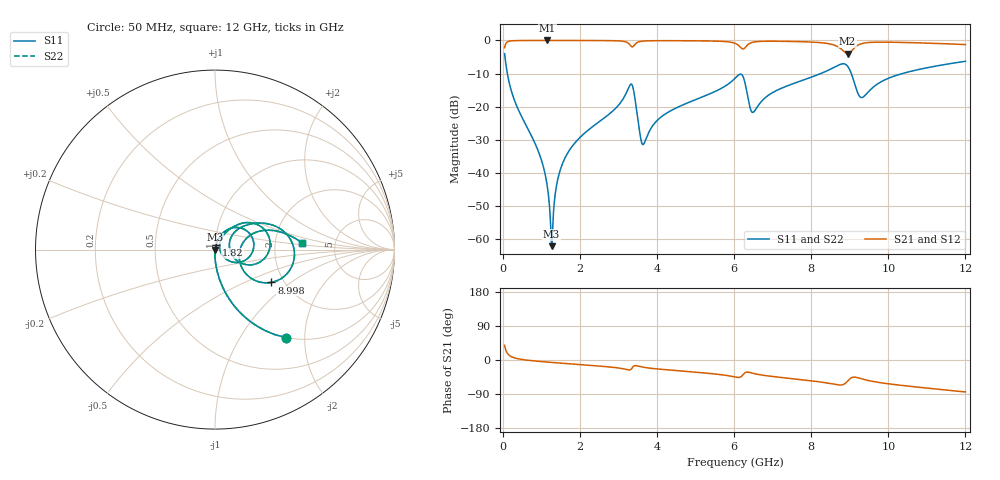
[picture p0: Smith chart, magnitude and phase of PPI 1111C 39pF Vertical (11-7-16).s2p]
# GHz S MA R 50
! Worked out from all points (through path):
!   1601 points, 50 MHz to 12 GHz, reference 50 ohm
!   highest |S21| = -0.01 dB at 1.155 GHz (marker M1); lowest = -4.0 dB at 8.945 GHz (marker M2)
!   group delay of S21, straight-line fit = 19.3 ps
!   lowest |S11| = -62.2 dB at 1.267 GHz (marker M3), VSWR 1.00, Z = 50.1 - j0.0248 ohm
!   |S11| at or under -10 dB: 120.9 MHz to 8.25 GHz (8.129 GHz wide, 194 % of centre); 9.041 GHz to 10.37 GHz (1.325 GHz wide, 13.7 % of centre)
!   |S22| runs from -62.2 to -4.0 dB; largest |S21 - S12| = 0
!   S11 on the Smith chart (normalised r, x): 50 MHz: 0.99, -1.62; 1.82 GHz: 1.01, +0.05; 8.998 GHz: 1.72, -0.73; 12 GHz: 2.84, +0.29
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0.05  0.6301 -51.2  0.7763 38.8  0.7763 38.8  0.6301 -51.2
0.2367188  0.1637 -81.6  0.9861 8.2  0.9861 8.2  0.1637 -81.6
0.9387813  0.02011 -91.7  0.9991 -3.6  0.9991 -3.6  0.02011 -91.7
1.155375  0.006347 -88.9  0.9992 -5.5  0.9992 -5.5  0.006347 -88.9
1.267406  0.0007793 -18.6  0.9992 -6.4  0.9992 -6.4  0.0007793 -18.6
1.469062  0.009927 77.2  0.999 -8.0  0.999 -8.0  0.009927 77.2
1.820094  0.02592 77.2  0.9986 -10.7  0.9986 -10.7  0.02592 77.2
2.044156  0.036 75.8  0.9981 -12.4  0.9981 -12.4  0.036 75.8
3.313844  0.2164 20.5  0.8374 -25.6  0.8374 -25.6  0.2164 20.5
3.396  0.1749 -20.5  0.8253 -16.3  0.8253 -16.3  0.1749 -20.5
3.627531  0.02683 5.1  0.9752 -18.8  0.9752 -18.8  0.02683 5.1
4.038312  0.06435 60.0  0.9908 -23.8  0.9908 -23.8  0.06435 60.0
6.025  0.2677 32.4  0.9055 -44.8  0.9055 -44.8  0.2677 32.4
6.219188  0.2947 -4.6  0.7459 -40.5  0.7459 -40.5  0.2947 -4.6
6.495531  0.08193 11.2  0.9414 -35.2  0.9414 -35.2  0.08193 11.2
8.019156  0.2806 31.8  0.9438 -55.0  0.9438 -55.0  0.2806 31.8
8.609188  0.3963 14.8  0.8457 -64.3  0.8457 -64.3  0.3963 14.8
8.945281  0.4083 -22.4  0.6331 -55.8  0.6331 -55.8  0.4083 -22.4
8.997563  0.3633 -30.2  0.6503 -50.2  0.6503 -50.2  0.3633 -30.2
9.303781  0.1371 -8.4  0.8921 -49.5  0.8921 -49.5  0.1371 -8.4
10.01331  0.2695 22.5  0.9412 -62.9  0.9412 -62.9  0.2695 22.5
12  0.4841 4.6  0.8658 -84.4  0.8658 -84.4  0.4841 4.6
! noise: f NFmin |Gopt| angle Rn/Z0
0.05  0.0003308  0.8511  0.8612  0.0004735
1.372  0.003262  0.634  6.902  0.001671
2.701  0.008566  0.7145  13.35  0.005846
4.031  0.01618  0.7704  20  0.01393
5.36  0.01777  0.7331  26.08  0.01262
6.682  0.03951  0.8444  32.6  0.04969
8.012  0.03356  0.7925  38.25  0.02984
9.341  0.0873  0.9041  44.47  0.171
10.67  0.03431  0.7525  49.19  0.02322
12  0.03072  0.7094  53.49  0.01672
